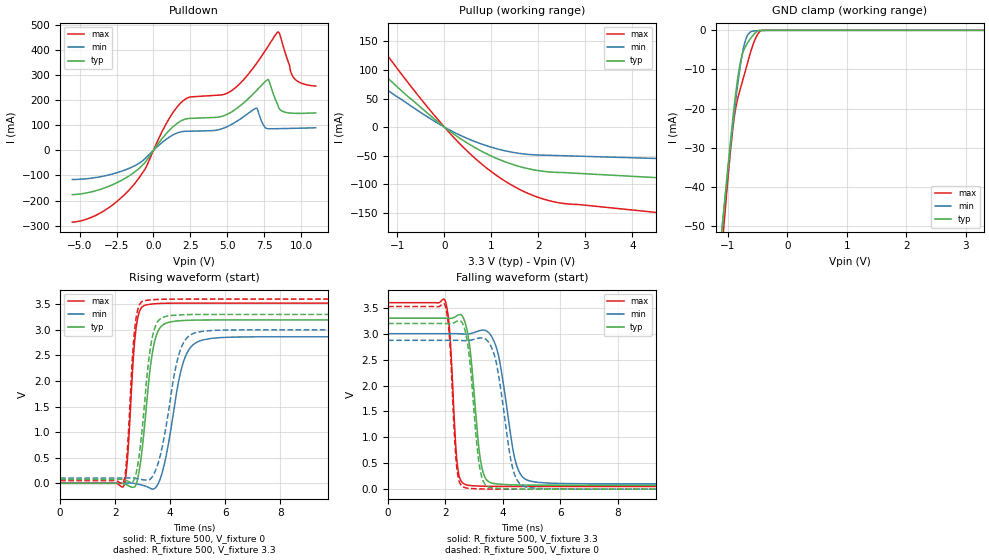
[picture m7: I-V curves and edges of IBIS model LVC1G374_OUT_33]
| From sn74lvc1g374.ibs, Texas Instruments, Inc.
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[Model]   LVC1G374_OUT_33
Model_type  3-state
Enable   Active-Low
Vref =   0
Rref =   500
Cref =   50p
Vmeas =   1.5
| variable   typ   min   max
C_comp   5.29pF   4.46pF   6.45pF
| C_pullup   8.11pF   5.29pF   9.38pF
| C_pulldown   8.23pF   5.99pF   11.74pF
| C_tri-state   5.29pF   4.46pF   6.45pF
[Temperature Range]   40   100   -40
| Ambient temperature   25   85   -40
[Voltage range]   3.3   3   3.6
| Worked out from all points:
|   slope of the pulldown table from 0 to 0.495 V, typ, clamps not added: 12.4 ohm
|   slope of the pullup table from 0 to 0.495 V, typ, clamps not added: 17.5 ohm
|   GND clamp passes 1 mA (typ) near -0.56 V on its own axis
|   rising waveform, R_fixture 500, V_fixture 0: 20-80 % time 381ps typ, 571ps min, 240ps max; typ from 0 V to 3.19 V
|   falling waveform, R_fixture 500, V_fixture 3.3: 20-80 % time 314ps typ, 477ps min, 201ps max; typ from 3.3 V to 0.076 V
|   rising waveform, R_fixture 500, V_fixture 3.3: 20-80 % time 371ps typ, 570ps min, 233ps max; typ from 0.076 V to 3.3 V
|   falling waveform, R_fixture 500, V_fixture 0: 20-80 % time 306ps typ, 456ps min, 196ps max; typ from 3.2 V to 0 V
[GND Clamp]
| LVC1G374_OUT_33
|   Voltage   I(typ)   I(min)   I(max)
-5.5V     -897.8mA   -832.4mA   -1.016A
-1.095V   -50.33mA   -50.14mA   -55.16mA
-1.065V   -45.41mA   -45.59mA   -49.63mA
-980mV    -31.93mA   -33.06mA   -34.73mA
-915mV    -22.35mA   -24.01mA   -24.95mA
-860mV    -15.14mA   -16.88mA   -19.23mA
-790mV    -8.202mA   -8.982mA   -14.91mA
-735mV    -5.197mA   -4.32mA    -11.95mA
-675mV    -3.353mA   -1.432mA   -8.641mA
-555mV    -899.1uA   -138.8uA   -2.764mA
-450mV    -10.12uA   -45.73uA   -166.1uA
3.3V      23.73pA    98.36nA    634.7pA
[Pulldown]
| LVC1G374_OUT_33
|   Voltage   I(typ)   I(min)   I(max)
-5.5V     -176.6mA   -116.3mA   -286.2mA
-3.535V   -154.2mA   -104.5mA   -247.3mA
-1.575V   -98.96mA   -70.04mA   -153.2mA
-565mV    -47.72mA   -32.93mA   -74.45mA
875mV     66.9mA     44.33mA    107mA
1.975V    120.1mA    74.7mA     195.4mA
5.04V     144.4mA    95.25mA    228.5mA
6.95V     235.6mA    167.2mA    342.7mA
7.74V     281.2mA    86.12mA    411.2mA
8.42V     182.5mA    86.1mA     470.1mA
9.48V     147.2mA    87.47mA    290.7mA
11V       148.7mA    89.5mA     255.6mA
[Pullup]
| LVC1G374_OUT_33
|   Voltage   I(typ)   I(min)   I(max)
-5.5V     471.4mA    370.4mA    661.1mA
-2.88V    227.2mA    175.2mA    323.5mA
-2.265V   173.3mA    132.6mA    248.1mA
-1.705V   126.1mA    95.63mA    181.7mA
-1.6V     117.5mA    88.94mA    169.5mA
-290mV    19.49mA    14.29mA    28.08mA
535mV     -30.29mA   -21.51mA   -45.84mA
1.35V     -62.49mA   -42.42mA   -97.53mA
1.815V    -73.33mA   -47.94mA   -117.2mA
2.205V    -78.19mA   -49.23mA   -128.2mA
7.355V    -101.1mA   -61.72mA   -173.1mA
11V       -117.5mA   -70.57mA   -203.8mA
[Ramp]
| LVC1G374_OUT_33
| variable   typ   min   max
dV/dt_r   1.96/3.96E-10   1.79/5.96E-10   2.16/2.51E-10
dV/dt_f   1.98/3.30E-10   1.78/4.99E-10   2.17/2.11E-10
R_load = 500
[Rising Waveform]
| LVC1G374_OUT_33
R_fixture =   500
C_fixture =   0
L_fixture =   0
V_fixture =   0
V_fixture_min = 0
V_fixture_max = 0
|   Time   V(typ)   V(min)   V(max)
0s        153.9pV    4.634nV    1.846nV
2.315ns   -8.296mV   862.3uV    -48.99mV
2.45ns    -36.95mV   4.292mV    492.6mV
2.75ns    -41.28mV   -6.767mV   2.978V
3.09ns    1.23V      -53.86mV   3.481V
3.335ns   2.482V     -112.1mV   3.502V
3.595ns   3.009V     26.71mV    3.513V
4.475ns   3.181V     2.356V     3.521V
5.215ns   3.191V     2.804V     3.521V
24.99ns   3.192V     2.864V     3.521V
[Falling Waveform]
| LVC1G374_OUT_33
R_fixture =   500
C_fixture =   0
L_fixture =   0
V_fixture =   3.3
V_fixture_min = 3
V_fixture_max = 3.6
|   Time   V(typ)   V(min)   V(max)
0s        3.3V       3V         3.6V
1.99ns    3.299V     3V         3.634V
2.15ns    3.295V     3V         3.025V
2.41ns    3.353V     3V         494.6mV
2.72ns    3.146V     2.993V     84.24mV
3.225ns   547.3mV    3.064V     58.81mV
3.615ns   117.4mV    2.94V      54.52mV
4.45ns    82.08mV    515.4mV    52.49mV
4.975ns   78.08mV    152.2mV    52.26mV
24.99ns   75.85mV    101.7mV    52.11mV
[Rising Waveform]
| LVC1G374_OUT_33
R_fixture =   500
C_fixture =   0
L_fixture =   0
V_fixture =   3.3
V_fixture_min = 3
V_fixture_max = 3.6
|   Time   V(typ)   V(min)   V(max)
0s        75.82mV    101.6mV    52.09mV
2.29ns    71.42mV    102.1mV    2.796mV
2.42ns    49.28mV    105.1mV    485.8mV
2.73ns    124.6mV    96.37mV    3.101V
3.06ns    1.496V     65.97mV    3.569V
3.275ns   2.617V     79.53mV    3.583V
3.515ns   3.128V     314.4mV    3.592V
4.32ns    3.29V      2.517V     3.599V
4.98ns    3.298V     2.951V     3.6V
24.99ns   3.3V       3V         3.6V
[Falling Waveform]
| LVC1G374_OUT_33
R_fixture =   500
C_fixture =   0
L_fixture =   0
V_fixture =   0
V_fixture_min = 0
V_fixture_max = 0
|   Time   V(typ)   V(min)   V(max)
0s        3.197V     2.871V     3.525V
1.98ns    3.197V     2.871V     3.555V
2.145ns   3.193V     2.871V     2.9V
2.395ns   3.24V      2.872V     416.5mV
2.705ns   3.012V     2.865V     25.95mV
3.185ns   442.9mV    2.917V     5.541mV
3.575ns   29.76mV    2.771V     1.956mV
4.34ns    4.764mV    408.8mV    359.2uV
4.815ns   1.721mV    41.54mV    161.8uV
24.99ns   27.83uV    40.13uV    18.38uV
